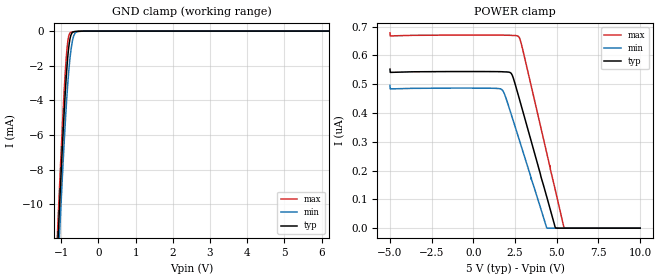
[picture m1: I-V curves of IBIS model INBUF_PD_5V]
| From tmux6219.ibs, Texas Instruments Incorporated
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| Model1
[Model]   INBUF_PD_5V
Model_type   Input
Vinl = 0.8
Vinh = 1.3
|   typ   min   max
C_comp   1.85pF   1.7pF   2.1pF
[Voltage Range]   5   4.5   5.5
[Temperature Range]   27   130   -40
[Power Clamp Reference]   5   4.5   5.5
[GND Clamp Reference]   0   0   0
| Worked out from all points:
|   GND clamp passes 1 mA (typ) near -0.80 V on its own axis
[GND Clamp]
|   Voltage   I(typ)   I(min)   I(max)
-5V       -219.2mA   -219.4mA   -219.1mA
-1.115V   -13.38mA   -14.94mA   -12.33mA
-1.07V    -11.23mA   -12.85mA   -10.14mA
-1.04V    -9.827mA   -11.48mA   -8.704mA
-950mV    -5.828mA   -7.568mA   -4.633mA
-875mV    -2.951mA   -4.671mA   -1.814mA
-815mV    -1.261mA   -2.762mA   -465.4uA
-740mV    -229.6uA   -1.106mA   -69.59uA
-695mV    -69.07uA   -517.3uA   -46.5uA
-635mV    -25.39uA   -138.4uA   -33.33uA
-410mV    -1.45uA    -2.381uA   -2.153uA
10V       0A         0A         0A
[POWER Clamp]
|   Voltage   I(typ)   I(min)   I(max)
-5V       552.6nA    496.3nA    678.5nA
-4.985V   541.2nA    483.9nA    667.9nA
1.675V    543.6nA    482.7nA    670.7nA
1.9V      543nA      460.7nA    670.5nA
2.275V    537.1nA    394.3nA    669.9nA
2.68V     464.6nA    319.9nA    667nA
2.785V    443nA      300.5nA    657.7nA
2.98V     402.8nA    264.5nA    615.1nA
4.39V     110.6nA    2.085nA    263nA
4.915V    815.7pA    0A         131.5nA
5.455V    0A         0A         0A
10V       0A         0A         0A
